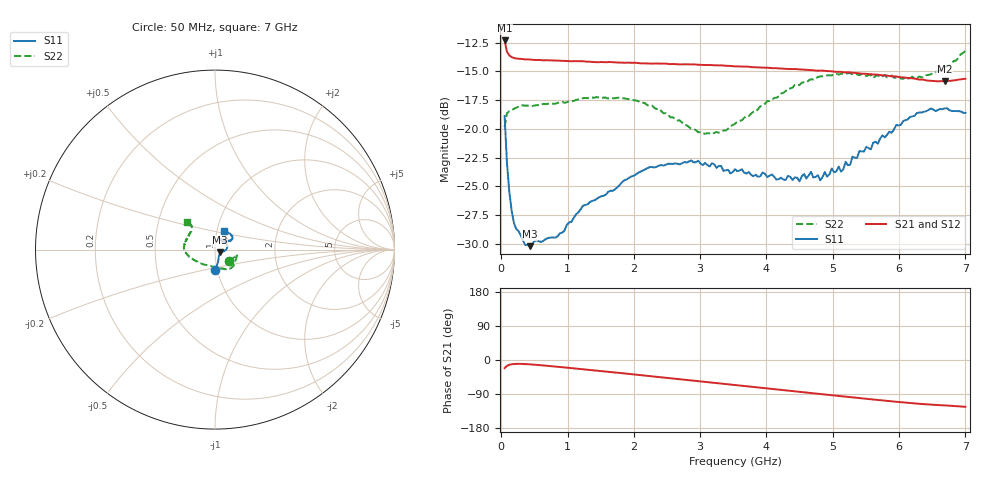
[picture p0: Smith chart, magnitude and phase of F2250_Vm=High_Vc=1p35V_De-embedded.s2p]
! Integrated Device Technology
! Corporate Headquarters
! 6024 Silver Creek Valley Road
! San Jose, CA 95138  USA
! Phone:  1-408-284-8200
! Toll Free:  1-800-223-1366
! Webpage:  http://www.idt.com/
! Timing and RF Division
! 515 Groton Road, Suite 102
! Westford, MA 01886-6024
! Device:  F2250
! Description: Voltage Variable RF Attenuator
! Frequency:  50.0 -  6000.00 MHz
! Package:  3x3 mm Thin QFN Plastic Package: 16 pin
! Ports:  2 RF, 3 DC
!  Pin  1  = GND
!  Pin  2  = NC
!  Pin  3  = RF1  = Port 1
!  Pin  4  = NC
!  Pin  5  = GND
!  Pin  6  = GND
!  Pin  7  = GND
!  Pin  8  = GND
!  Pin  9  = NC
!  Pin 10  = RF2  = Port 2
!  Pin 11  = NC
!  Pin 12  = GND
!  Pin 13  = GND
!  Pin 14  = VCNTRL
!  Pin 15  = VDD
!  Pin 16  = VMODE
! Vcntrl:  1.350 Volts
! Vmode:  +3.300 Volts
! Vdd:  +3.30  Volts
! Current:  1.333 mA
! Data:  The device was measured on a the F2250 evaluation board which has
!  individual transmission lines to the RF pins.  Data was collected
!  using a calibrated network analyzer.  The evaluation board was
!  de-embedded using a TRL calibration technique.
!  The reference plane is the edge of the package pin.
! Misc:  SN 10
!  Action Tracker AT0258
! Date Measured:  2014-11-26
! Date:  2015-10-15  MJV
! Note:
!  Integrated Device Technology supplies this data as a sample of measured
!  data at the package pin for this product.  Your particular data for this
!  product may vary.
!  Data was taken at 25 degrees C.
!  Integrated Device Technology reserves the right to change this data at anytime.
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# GHz S dB R 50
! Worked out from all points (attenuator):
!   201 points, 50 MHz to 7 GHz, reference 50 ohm
!   highest |S21| = -12.31 dB at 50 MHz (marker M1); lowest = -15.9 dB at 6.687 GHz (marker M2)
!   lowest |S11| = -30.2 dB at 432.2 MHz (marker M3), VSWR 1.06, Z = 52.7 - j1.59 ohm
!   |S11| at or under -10 dB: start of sweep to end of sweep
!   |S22| runs from -20.5 to -13.2 dB; largest |S21 - S12| = 0.00079
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0.05  -18.88 -90.1  -12.31 -21.4  -12.32 -21.4  -19.86 -39.0
0.08475  -22.90 -75.9  -13.29 -15.5  -13.27 -15.5  -18.66 -20.3
0.1195  -25.40 -68.4  -13.61 -12.7  -13.60 -12.7  -18.47 -15.1
0.189  -28.16 -54.2  -13.83 -10.5  -13.81 -10.5  -18.26 -13.3
0.43225  -30.21 -29.1  -13.98 -11.5  -13.98 -11.5  -18.00 -16.0
0.84925  -29.36 -17.8  -14.07 -17.9  -14.05 -17.9  -17.75 -29.4
1.2315  -26.70 -14.4  -14.12 -24.4  -14.13 -24.5  -17.33 -39.2
2.37825  -23.20 10.8  -14.32 -44.8  -14.33 -44.9  -18.26 -63.6
3.07325  -22.98 32.5  -14.45 -57.7  -14.46 -57.7  -20.45 -97.7
3.525  -23.53 48.6  -14.57 -66.0  -14.56 -66.0  -19.57 -129.0
4.1505  -24.42 65.1  -14.72 -77.5  -14.74 -77.5  -17.30 -158.6
4.498  -24.58 62.6  -14.82 -84.0  -14.83 -84.0  -16.18 -169.4
4.67175  -23.75 61.7  -14.90 -87.2  -14.90 -87.2  -15.69 -173.1
4.7065  -24.23 62.3  -14.91 -87.8  -14.92 -87.8  -15.71 -173.7
5.1235  -23.72 49.4  -15.04 -95.5  -15.06 -95.5  -15.22 177.0
5.193  -22.87 44.7  -15.10 -96.7  -15.08 -96.8  -15.24 175.8
5.2625  -23.11 40.7  -15.10 -98.0  -15.10 -98.0  -15.17 174.7
5.29725  -22.42 40.3  -15.12 -98.6  -15.12 -98.7  -15.26 173.7
5.85325  -20.25 31.0  -15.41 -108.4  -15.41 -108.6  -15.50 159.1
6.27025  -18.63 33.0  -15.68 -115.1  -15.68 -115.2  -15.60 145.9
6.68725  -18.22 45.0  -15.87 -119.8  -15.89 -119.9  -14.65 134.6
7  -18.62 64.8  -15.65 -123.5  -15.65 -123.7  -13.19 134.6
